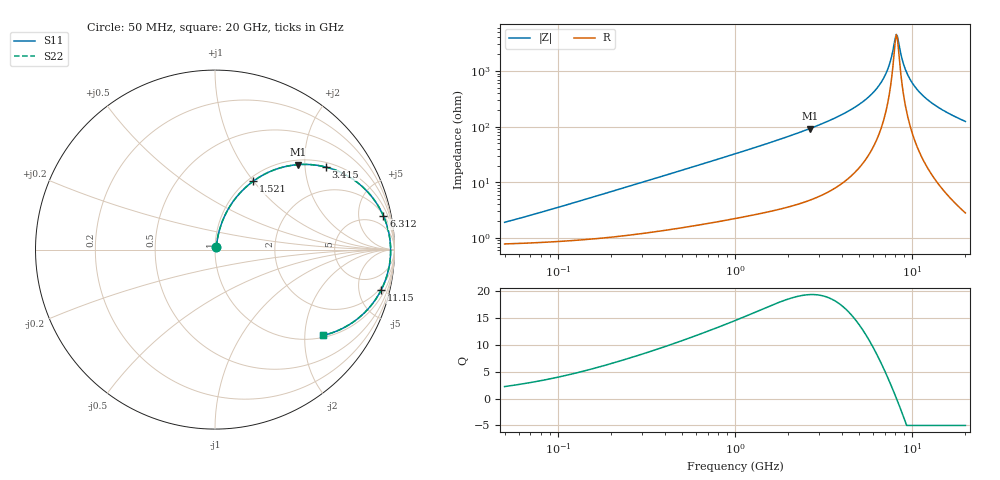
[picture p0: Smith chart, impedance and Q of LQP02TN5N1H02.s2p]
!Murata Part Number: LQP02TN5N1H02
!These Parameters are Measured in Series Mode Connection
!  o--[Z]--o
!Port1  Port2
!  o-------o
!Freq. Start=50[MHz] Stop=20[GHz], 401[Steps]
# Hz S RI R 50
!Freq.(Hz) S11(Real) S11(Imag) S21(Real) S21(Imag) S12(Real) S12(Imag) S22(Real) S22(Imag)
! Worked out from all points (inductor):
!   401 points, 50 MHz to 20 GHz, reference 50 ohm
!   read as one part in series: L = 5.48 nH near 70.56 MHz
!   highest Q = 19.3 at 2.647 GHz (marker M1), where L = 5.54 nH
!   self-resonance near 8.142 GHz
!   S11 on the Smith chart (normalised r, x): 50 MHz: 1.02, +0.03; 1.521 GHz: 1.06, +0.99; 3.415 GHz: 1.14, +2.57; 6.312 GHz: 2.16, +9.59; 11.15 GHz: 1.63, -7.95; 20 GHz: 1.06, -2.48
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5e7  0.00804 0.0172  0.992 -0.0172  0.992 -0.0172  0.00804 0.0172
1.364002e8  0.0112 0.0455  0.9888 -0.0455  0.9888 -0.0455  0.0112 0.0455
3.721004e8  0.0273 0.1178  0.9727 -0.1178  0.9727 -0.1178  0.0273 0.1178
1e9  0.1108 0.2813  0.8892 -0.2813  0.8892 -0.2813  0.1108 0.2813
1.521052e9  0.2116 0.3801  0.7884 -0.3801  0.7884 -0.3801  0.2116 0.3801
2.647493e9  0.4621 0.4734  0.5379 -0.4734  0.5379 -0.4734  0.4621 0.4734
2.728004e9  0.4795 0.4744  0.5205 -0.4744  0.5205 -0.4744  0.4795 0.4744
3.415248e9  0.6178 0.4599  0.3822 -0.4599  0.3822 -0.4599  0.6178 0.4599
4.89267e9  0.8318 0.3406  0.1682 -0.3406  0.1682 -0.3406  0.8318 0.3406
5.598765e9  0.8951 0.2656  0.1049 -0.2656  0.1049 -0.2656  0.8951 0.2656
6.311513e9  0.9381 0.1881  0.0619 -0.1881  0.0619 -0.1881  0.9381 0.1881
6.905011e9  0.9607 0.1248  0.0393 -0.1248  0.0393 -0.1248  0.9607 0.1248
7.442007e9  0.9727 0.0698  0.0273 -0.0698  0.0273 -0.0698  0.9727 0.0698
8.020766e9  0.9782 0.0135  0.0218 -0.0135  0.0218 -0.0135  0.9782 0.0135
8.264682e9  0.9785 -0.00909  0.0215 0.00909  0.0215 0.00909  0.9785 -0.00909
8.389408e9  0.9783 -0.0204  0.0217 0.0204  0.0217 0.0204  0.9783 -0.0204
8.907419e9  0.9748 -0.0656  0.0252 0.0656  0.0252 0.0656  0.9748 -0.0656
9.316812e9  0.9694 -0.0991  0.0306 0.0991  0.0306 0.0991  0.9694 -0.0991
1.004137e10  0.9551 -0.1539  0.0449 0.1539  0.0449 0.1539  0.9551 -0.1539
1.115139e10  0.9249 -0.2268  0.0751 0.2268  0.0751 0.2268  0.9249 -0.2268
1.438523e10  0.8083 -0.3741  0.1917 0.3741  0.1917 0.3741  0.8083 -0.3741
2e10  0.6037 -0.4779  0.3963 0.4779  0.3963 0.4779  0.6037 -0.4779
